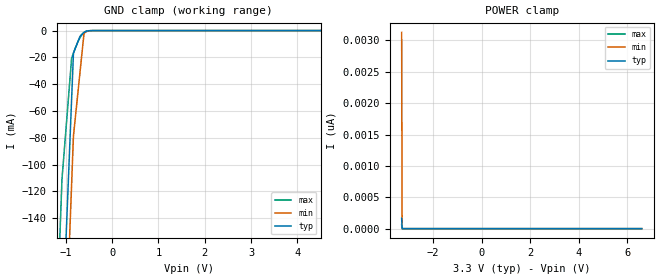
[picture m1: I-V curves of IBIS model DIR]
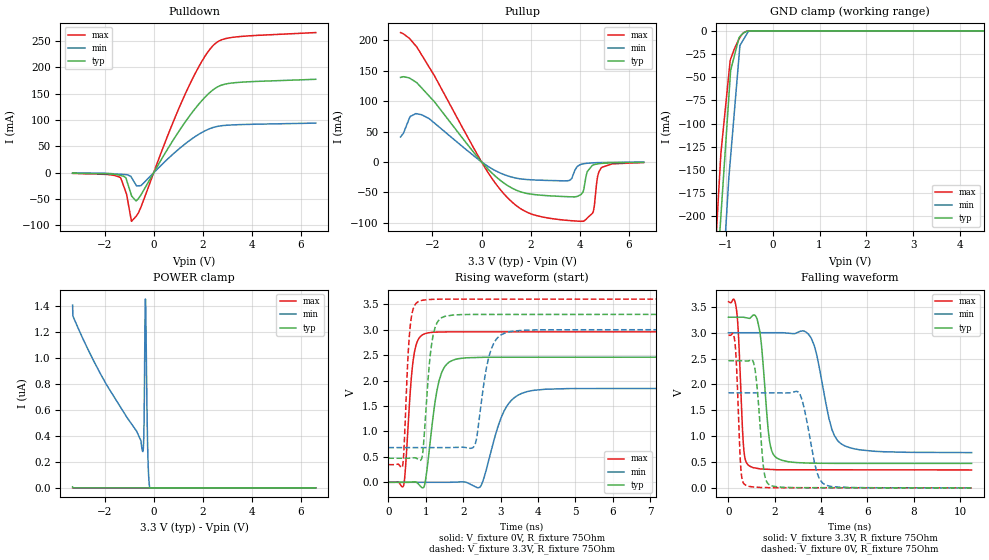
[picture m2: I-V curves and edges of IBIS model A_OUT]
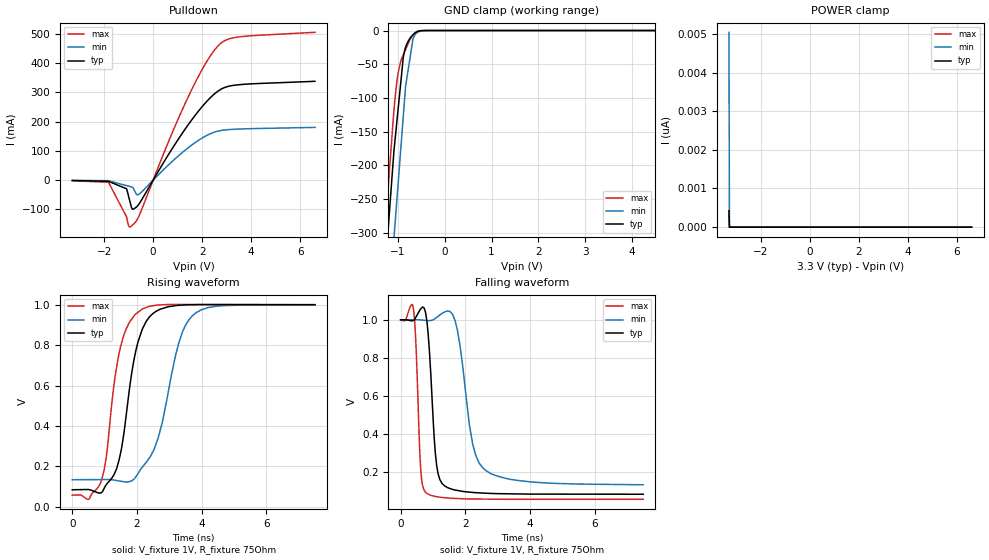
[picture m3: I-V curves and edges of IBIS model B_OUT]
| Texas Instruments Incorporated
| 4-bits LVTTL to GTL Transceiver
| Marketing part#   Voltage Range   Package-type   #pins/pkg drawing
| SN74GTL2014PW   3.0V - 3.6V   TSSOP   14-pin PW
[IBIS Ver]   4.1
[File name]   sn74gtl2014.ibs
[File Rev]   1.0
[Date]   11/06/2013
[Source]   Model built from spectre simulations at:
   Texas Instruments Incorporated.
   Analog-eLab, HPA
   12500 TI Blvd
   Dallas, TX -75243
   For Support e-mail: elab_ibis@list.ti.com
[Notes]   Revision History
   Rev 1.0: 11/06/2013
   - ccomp values are based on PVT settings:
   MIN: Low Voltage, High Temperature, Weak Process
   TYP: Nominal Voltage, Nominal Temperature, Nominal Process
   MAX: High Voltage, Low Temperature, Fast Process
   - C_comp although listed in numerical order of value are obtained from varying PVT conditions.
   For PVT conditions for each specific value, refer to the buffer description under respective [Model].
   IBIS model user is responsible for using appropriate C_comp to simulate for Signal Integrity.
[Disclaimer]  This model is designed as an aid for customers of Texas Instruments
 TI and its licensors and suppliers make no warranties, either expressed
 or implied, with respect to this  model, including the warranties of
 merchantability or fitness for a particular purpose.
 The model is provided solely on an "as is" basis. The entire risk as to
 its quality and performance is with the customer.
[Copyright] (C)Copyright 2013 Texas Instruments Incorporated.
   All rights reserved.
[Component]   GTL2014
[Manufacturer]  Texas Instruments Incorporated
[Package]   |14-pin PW package
|   typ   min   max
R_pkg   0   0   0
L_pkg   0   0   0
C_pkg   0   0   0
[Pin]   signal_name   model_name   R_pin   L_pin   C_pin
1   DIR   DIR   0.14018  2.92565n  0.39967p
2   B0   B_OUT   0.15023  2.32850n  0.31410p
3   B1   B_OUT   0.13516  2.14548n  0.30509p
4   VREF   NC   0.11455  1.90000n  0.29171p
5   B2   B_OUT   0.11176  1.86771n  0.28896p
6   B3   B_OUT   0.11064  1.85626n  0.28880p
7   GND   GND   0.09790  2.42689n  0.37387p
8   GND   GND   0.10060  2.45412n  0.37507p
9   A3   B_OUT   0.11064  1.85080n  0.28821p
10   A2   B_OUT   0.11176  1.86078n  0.28876p
11   GND   GND   0.11455  1.89328n  0.29154p
12   A1   B_OUT   0.13516  2.13981n  0.30510p
13   A0   B_OUT   0.15023  2.32455n  0.31688p
14   VCC1   POWER   0.07569  2.57781n  0.43723p
| Models and submodels in the file (3): DIR (Input), A_OUT (I/O), B_OUT (I/O_open_drain)
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|   (nom PVT)   (slow PVT)   (fast PVT)
|   Model SCK
[Model]   DIR
Model_type   Input
Vinl = .8
Vinh = 2
|   typ   min   max
C_comp   1.756p   1.749p   1.767p
|C_comp (ON state)   1.000e-200   NA   NA
|C_comp (OFF state)   1.000e-200   NA   NA
[Voltage Range]   3.3   3   3.6
[Temperature Range]   27   125   -40
[Power Clamp Reference]   3.3   3   3.6
[GND Clamp Reference]   0   0   0
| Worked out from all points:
|   GND clamp passes 1 mA (typ) near -0.59 V on its own axis
[GND Clamp]
|   Voltage   I(typ)   I(min)   I(max)
-3.3V     -2.323A    -2.424A    -2.261A
-1.825V   -873.2mA   -980mA     -807.1mA
-1.082V   -231mA     -304mA     -111mA
-874.5mV  -51.16mA   -114.8mA   -20.8mA
-834.9mV  -16.91mA   -78.71mA   -16.77mA
-765.6mV  -10.71mA   -55.43mA   -10.59mA
-696.3mV  -4.503mA   -32.14mA   -5.542mA
-607.2mV  -1.414mA   -2.207mA   -1.438mA
-567.6mV  -693.1uA   -1.052mA   -602.2uA
-488.4mV  -114.9uA   -222.9uA   -65.78uA
-330mV    -1.191uA   -6.641uA   -159.9nA
6.6V      0A         0A         0A
[POWER Clamp]
|   Voltage   I(typ)   I(min)   I(max)
-3.3V     167.3pA    3.129nA    63.65pA
-3.28V    0A         0A         0A
-3.27V    0A         0A         0A
6.6V      0A         0A         0A
|   Model A_OUT
[Model]   A_OUT
Model_type   I/O
Polarity   Non-Inverting
Enable   Active-Low
Vinl = .8
Vinh = 2
Vmeas = 1.65
Vref = 3.3
Cref = 15pF
Rref = 75
|   typ   min   max
C_comp   1.000e-200   NA   NA
|C_comp (ON state)   4.223p   4.135p   4.307p
|C_comp (OFF state)   3.637p   3.610p   3.865p
[Voltage Range]   3.3   3   3.6
[Temperature Range]   27   125   -40
[Pullup Reference]   3.3   3   3.6
[Pulldown Reference]   0   0   0
[Power Clamp Reference]   3.3   3   3.6
[GND Clamp Reference]   0   0   0
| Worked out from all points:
|   slope of the pulldown table from 0 to 0.495 V, typ, clamps not added: 12.6 ohm
|   slope of the pullup table from 0 to 0.495 V, typ, clamps not added: 23.5 ohm
|   GND clamp passes 1 mA (typ) near -0.57 V on its own axis
|   falling waveform, V_fixture 3.3V, R_fixture 75Ohm: 20-80 % time 307ps typ, 630ps min, 191ps max; typ from 3.3 V to 0.473 V
|   rising waveform, V_fixture 0V, R_fixture 75Ohm: 20-80 % time 276ps typ, 490ps min, 173ps max; typ from 0 V to 2.46 V
|   rising waveform, V_fixture 3.3V, R_fixture 75Ohm: 20-80 % time 191ps typ, 304ps min, 131ps max; typ from 0.473 V to 3.3 V
|   falling waveform, V_fixture 0V, R_fixture 75Ohm: 20-80 % time 259ps typ, 480ps min, 160ps max; typ from 2.46 V to 0 V
[Pulldown]
|   Voltage   I(typ)   I(min)   I(max)
-3.3V     -779.9uA   -435.8uA   -1.14mA
-1.34V    -5.208mA   -2.849mA   -9.771mA
-1.102V   -13.82mA   -3.632mA   -40.63mA
-904.2mV  -42.95mA   -8.828mA   -92.06mA
-716.1mV  -53.44mA   -23.37mA   -82.7mA
-518.1mV  -42.03mA   -24.41mA   -65.13mA
1.125V    85.54mA    48.92mA    132.7mA
1.818V    129.1mA    72.47mA    199.6mA
2.393V    156.3mA    85.49mA    240mA
2.719V    165.5mA    88.94mA    251.3mA
3.204V    170.4mA    90.78mA    256.9mA
6.6V      177.3mA    94.2mA     266mA
[GND Clamp]
|   Voltage   I(typ)   I(min)   I(max)
-3.3V     -2.327A    -2.429A    -2.264A
-1.191V   -275.8mA   -389mA     -211.9mA
-1.132V   -222.6mA   -333mA     -158.8mA
-1.102V   -200.2mA   -304.9mA   -132.3mA
-1.003V   -125.2mA   -217.4mA   -82.15mA
-904.2mV  -50.23mA   -141.5mA   -32.01mA
-894.3mV  -42.74mA   -135.5mA   -30.42mA
-696.3mV  -6.196mA   -15.86mA   -7.141mA
-577.5mV  -1.136mA   -5.754mA   -944.7uA
-518.1mV  -317.9uA   -703.2uA   -195.1uA
-369.6mV  -5.426uA   -26.42uA   -1.026uA
6.6V      0A         0A         0A
[Pullup]
|   Voltage   I(typ)   I(min)   I(max)
-3.3V     139mA      41.1mA     212.9mA
-2.914V   137.5mA    74.54mA    202.1mA
-2.439V   121.7mA    77.64mA    176mA
293.7mV   -13.09mA   -8.12mA    -19.35mA
1.68V     -50.29mA   -28.39mA   -79.18mA
3.561V    -57.31mA   -30.57mA   -96.44mA
4.165V    -44.34mA   -2.946mA   -97.35mA
4.303V    -15.88mA   -2.191mA   -92.28mA
4.551V    -5.002mA   -1.49mA    -81.26mA
4.719V    -3.299mA   -1.221mA   -25.19mA
4.877V    -2.482mA   -1.042mA   -9.467mA
6.6V      -655.4uA   -397.1uA   -1.055mA
[POWER Clamp]
|   Voltage   I(typ)   I(min)   I(max)
-3.3V     7.282nA    1.408uA    907.7pA
-3.29V    3.641nA    1.326uA    453.9pA
-2.676V   0A         1.068uA    0A
-438.9mV  0A         279.5nA    0A
-399.3mV  0A         413.8nA    0A
-379.5mV  0A         689.7nA    0A
-349.8mV  0A         1.346uA    0A
-330mV    0A         1.453uA    0A
-250.8mV  0A         375.4nA    0A
-211.2mV  0A         118.9nA    0A
-161.7mV  0A         1.382nA    0A
6.6V      0A         0A         0A
[Ramp]
R_load = 75
|   typ   min   max
dV/dt_r   1.47537/2.75664e-10   1.1071/4.89179e-10   1.77413/1.72751e-10
dV/dt_f   1.69646/3.0719e-10   1.39083/6.30157e-10   1.95203/1.90246e-10
[Falling Waveform]
V_fixture = 3.3V
V_fixture_min = 3V
V_fixture_max = 3.6V
R_fixture = 75Ohm
C_fixture = 0F
|   Time   V(typ)   V(min)   V(max)
0s        3.3V       3V         3.6V
344ps     3.3V       3V         3.456V
665ps     3.299V     3V         730mV
917.4ps   3.279V     3V         421mV
1.358ns   3.021V     3V         367.4mV
1.768ns   927.6mV    3V         357.4mV
2.072ns   583.7mV    3.001V     350.7mV
3.576ns   478.2mV    2.895V     349.4mV
4.844ns   473.3mV    859.3mV    348.9mV
10.5ns    472.6mV    682mV      346.6mV
[Rising Waveform]
V_fixture = 0V
V_fixture_min = 0V
V_fixture_max = 0V
R_fixture = 75Ohm
C_fixture = 0F
|   Time   V(typ)   V(min)   V(max)
0s        243.8nV    87.58nV    369.1nV
408.9ps   -147.3uV   -102.7uV   -59.67mV
665ps     7.969mV    -167.1uV   2.407V
984.6ps   6.681mV    -247.5uV   2.923V
1.358ns   2.001V     -341.3uV   2.953V
1.768ns   2.411V     3.183mV    2.957V
2.477ns   2.455V     -67.94mV   2.957V
3.096ns   2.458V     1.403V     2.957V
3.709ns   2.458V     1.782V     2.957V
10.5ns    2.459V     1.845V     2.957V
[Rising Waveform]
V_fixture = 3.3V
V_fixture_min = 3V
V_fixture_max = 3.6V
R_fixture = 75Ohm
C_fixture = 0F
|   Time   V(typ)   V(min)   V(max)
0s        472.6mV    682mV      346.6mV
387.3ps   472.5mV    681.9mV    351.8mV
583.1ps   474.6mV    681.9mV    3.061V
808.6ps   443.7mV    681.8mV    3.554V
1.159ns   2.729V     681.8mV    3.595V
1.461ns   3.249V     681.7mV    3.599V
2.317ns   3.299V     740.2mV    3.599V
2.71ns    3.299V     2.521V     3.599V
3.153ns   3.299V     2.943V     3.599V
10.5ns    3.3V       3V         3.6V
[Falling Waveform]
|Gnd
V_fixture = 0V
V_fixture_min = 0V
V_fixture_max = 0V
R_fixture = 75Ohm
C_fixture = 0F
|   Time   V(typ)   V(min)   V(max)
0s        2.459V     1.838V     2.957V
283.7ps   2.459V     1.838V     2.8V
534.5ps   2.459V     1.838V     379.3mV
734.4ps   2.455V     1.837V     53.85mV
1.123ns   2.354V     1.837V     15.05mV
1.527ns   348.3mV    1.836V     6.549mV
1.768ns   59.58mV    1.836V     3.83mV
3.096ns   3.471mV    1.801V     2.447mV
4.196ns   2.955mV    55.79mV    2.084mV
10.5ns    243.8nV    287.4uV    369.1nV
|   Model B_OUT
[Model]   B_OUT
Model_type   I/O_open_drain
Polarity   Non-Inverting
Enable   Active-Low
Vinl = .4
Vinh = 2.4
Vmeas = 1.65
Vref = 3.3
Cref = 15pF
Rref = 75
|   typ   min   max
|   (nom PVT)   (Fast PVT)   (slow PVT)
C_comp   3.112p   3.088p   3.127p
|C_comp (ON state)   3.112p   3.088p   3.127p
|C_comp (OFF state)   3.352p   3.156p   3.902p
| Where   nom PVT is  Nominal Process, 3.3V, 27C
|   Fast PVT is Strong Process, 3.45V, -40C
|   Slow PVT is Weak Process, 3.15V, 125C
[Voltage Range]   3.3   3   3.6
[Temperature Range]   27   125   -40
[Pullup Reference]   3.3   3   3.6
[Pulldown Reference]   0   0   0
[Power Clamp Reference]   3.3   3   3.6
[GND Clamp Reference]   0   0   0
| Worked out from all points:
|   slope of the pulldown table from 0 to 0.495 V, typ, clamps not added: 7.1 ohm
|   GND clamp passes 1 mA (typ) near -0.56 V on its own axis
|   falling waveform, V_fixture 1V, R_fixture 75Ohm: 20-80 % time 196ps typ, 426ps min, 123ps max; typ from 1 V to 0.085 V
|   rising waveform, V_fixture 1V, R_fixture 75Ohm: 20-80 % time 540ps typ, 745ps min, 473ps max; typ from 0.085 V to 1 V
[Pulldown]
|   Voltage   I(typ)   I(min)   I(max)
-3.3V     -1.504mA   -834.7uA   -2.233mA
-1.825V   -4.284mA   -2.127mA   -7.325mA
-1.082V   -29.74mA   -18.94mA   -126.9mA
-993.3mV  -58.48mA   -20.96mA   -157.8mA
-933.9mV  -77.63mA   -22.31mA   -160.8mA
-834.9mV  -99.48mA   -24.55mA   -152.8mA
-607.2mV  -84.98mA   -49.58mA   -127.7mA
1.393V    184.8mA    108mA      277.7mA
2.095V    260.3mA    148.4mA    392.2mA
2.64V     303.7mA    167.2mA    458mA
3.472V    325.5mA    174.3mA    488.7mA
6.6V      337.4mA    180mA      504.7mA
[GND Clamp]
|   Voltage   I(typ)   I(min)   I(max)
-3.3V     -2.323A    -2.424A    -2.261A
-1.825V   -874mA     -980.8mA   -808.1mA
-1.085V   -180.5mA   -310mA     -119.6mA
-1.073V   -170.8mA   -298.3mA   -109.9mA
-1.063V   -164mA     -289.3mA   -102.8mA
-993.3mV  -115.8mA   -226.4mA   -62.36mA
-933.9mV  -74.59mA   -172.6mA   -44.01mA
-884.4mV  -40.21mA   -127.7mA   -36.13mA
-834.9mV  -24.93mA   -82.75mA   -28.24mA
-676.5mV  -6.158mA   -12.36mA   -6.733mA
-587.4mV  -1.703mA   -3.028mA   -1.412mA
6.6V      0A         0A         0A
[POWER Clamp]
|   Voltage   I(typ)   I(min)   I(max)
-3.3V     425.6pA    5.039nA    312.2pA
-3.28V    0A         0A         0A
-3.27V    0A         0A         0A
6.6V      0A         0A         0A
[Ramp]
R_load = 75
|   typ   min   max
dV/dt_r   0.549099/5.40165e-10   0.519325/7.44677e-10   0.565142/4.72601e-10
dV/dt_f   0.549099/1.96358e-10   0.519325/4.25619e-10   0.565142/1.22826e-10
[Falling Waveform]
V_fixture = 1V
V_fixture_min = 1V
V_fixture_max = 1V
R_fixture = 75Ohm
C_fixture = 0F
|   Time   V(typ)   V(min)   V(max)
0s        1V         1V         1V
386.4ps   995.6mV    999.9mV    1.068V
622ps     1.057V     999.1mV    213.5mV
819.8ps   980.1mV    996.3mV    88.29mV
1.115ns   234.8mV    1.012V     72.02mV
1.368ns   127.7mV    1.041V     66.62mV
1.687ns   106.8mV    993.4mV    62.84mV
2.226ns   94.29mV    348.6mV    59.74mV
2.533ns   91.05mV    224.1mV    59.3mV
7.5ns     84.84mV    134.5mV    58.1mV
[Rising Waveform]
V_fixture = 1V
V_fixture_min = 1V
V_fixture_max = 1V
R_fixture = 75Ohm
C_fixture = 0F
|   Time   V(typ)   V(min)   V(max)
0s        84.84mV    134.5mV    58.1mV
867.1ps   68.68mV    135.1mV    116.2mV
1.049ns   109.5mV    135.2mV    243.1mV
1.285ns   158mV      132.9mV    598.8mV
1.547ns   313.8mV    125.6mV    825.6mV
1.939ns   753.6mV    143.5mV    951.3mV
2.533ns   960.9mV    286mV      995.9mV
3.292ns   997.2mV    811.2mV    1.001V
3.693ns   1V         942.2mV    1.001V
7.5ns     1V         1V         1V
